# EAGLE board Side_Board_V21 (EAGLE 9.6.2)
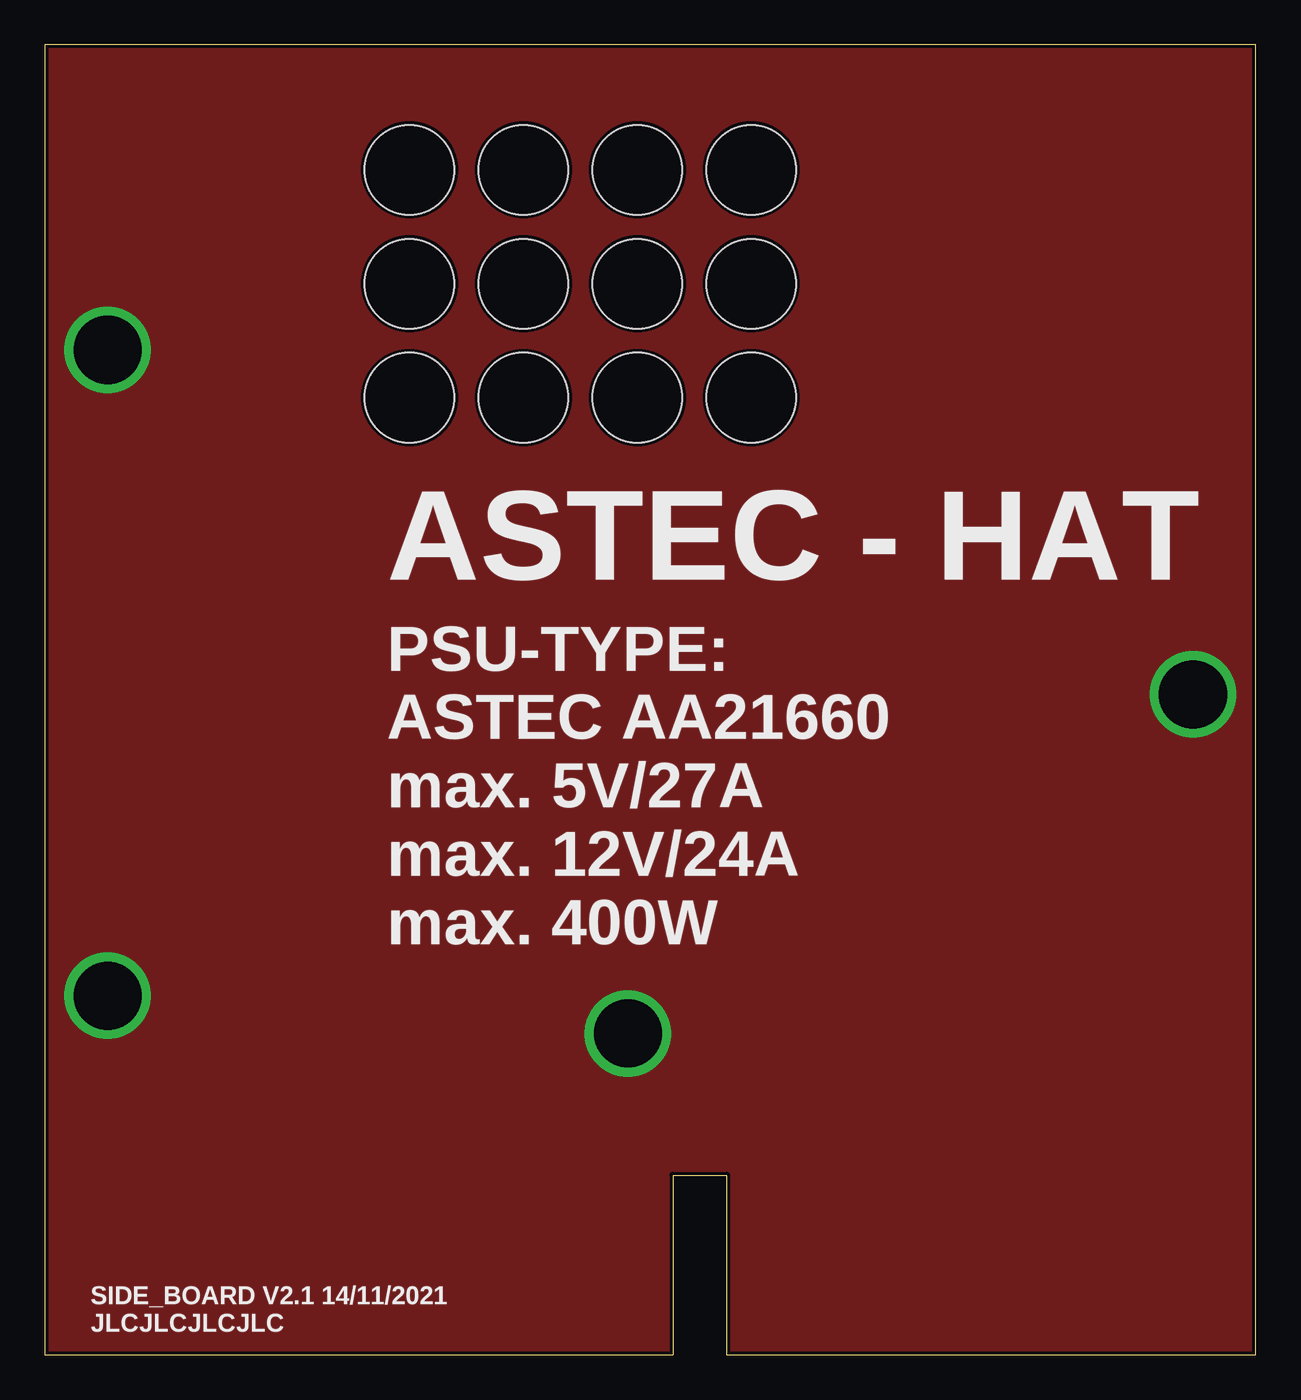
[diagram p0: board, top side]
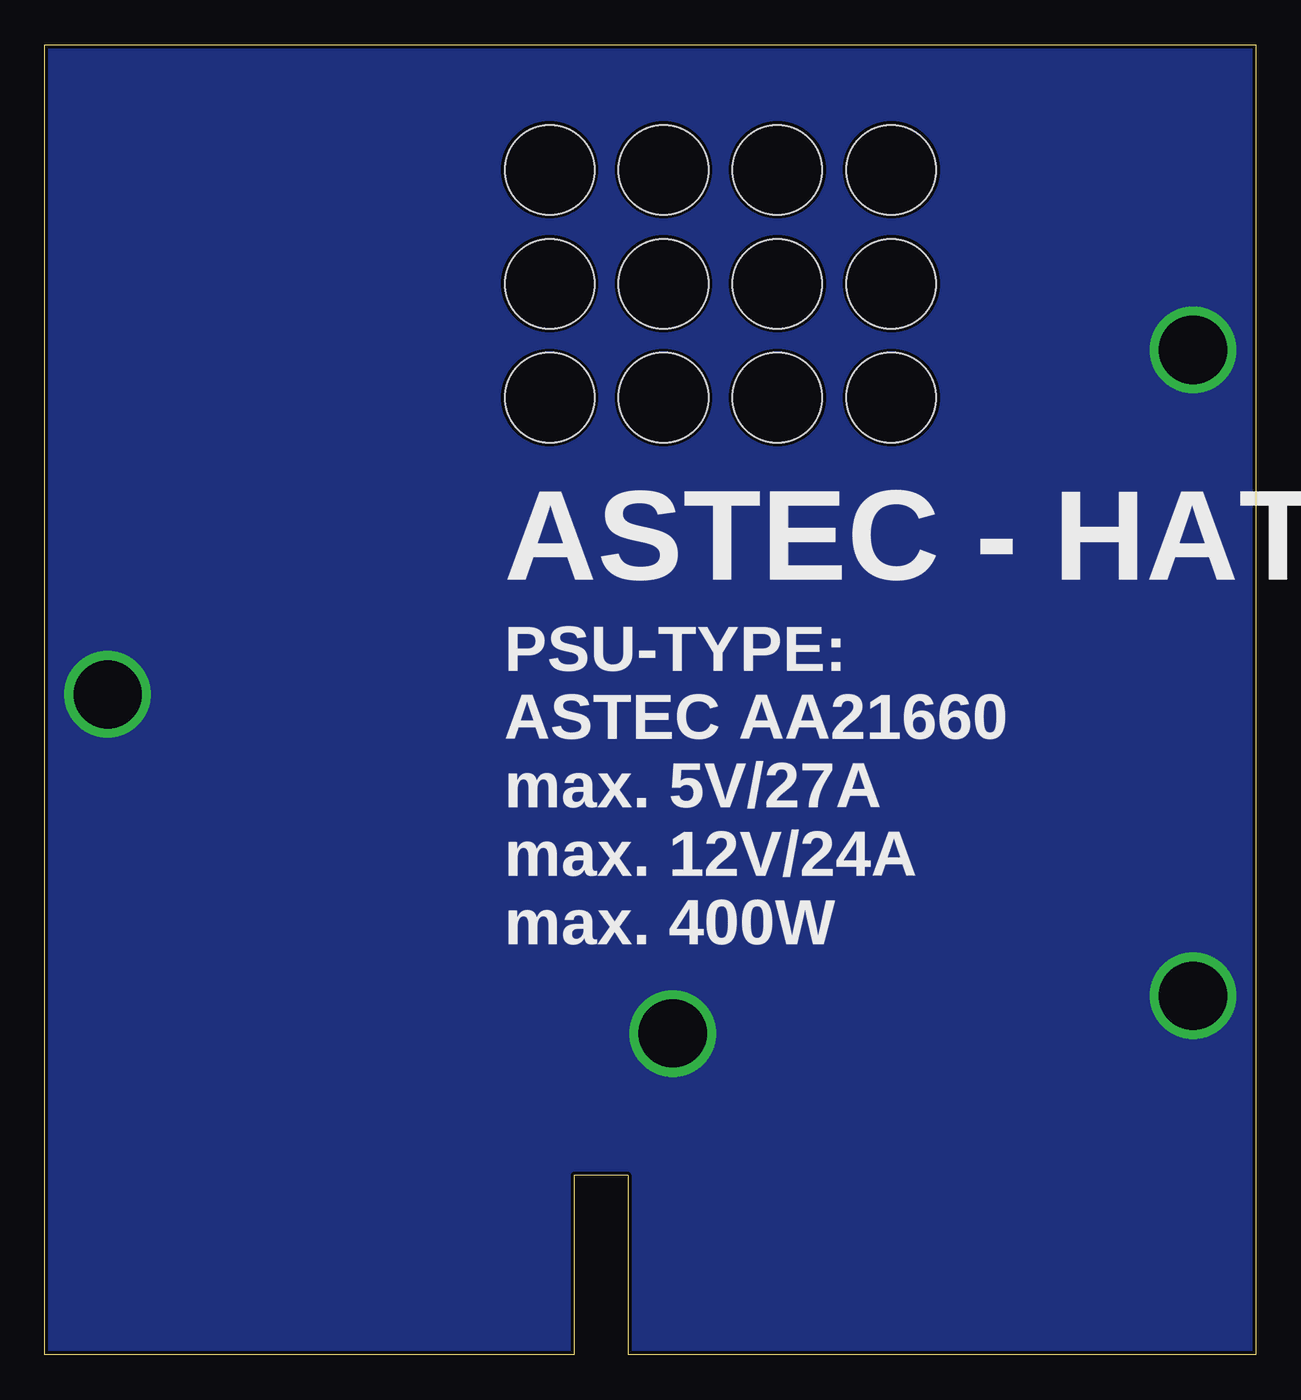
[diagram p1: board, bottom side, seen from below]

Size 67.5 x 73 mm. Coordinates in mm from the lower left corner, seen from the top.
Outline: 38,0 67.5,0 67.5,73 0,73 0,0 35,0 35,10 38,10 38,0
Copper layers (1*16): Top 0.035mm / dielectric 1.5mm / Bottom 0.035mm
Design rules "JLCPCB_2alyer": minimum track width 5mil, minimum drill 0.2mm, track to track 5mil, track to pad 0.2mm, pad to pad 0.2mm, via to via 0.2mm, smd to smd 5mil, copper to edge 0.2mm, drill to drill 0.5mm, minimum pad ring 0.13mm, minimum via ring 0.13mm, stop-mask expansion 0.05mm, vias tented up to drill 0mil, thermal gap 10mil
Holes 5 mm at 20.32,66.04 26.67,66.04 33.02,66.04 39.37,66.04 20.32,59.69 20.32,53.34 26.67,59.69 33.02,59.69 26.67,53.34 33.02,53.34 39.37,59.69 39.37,53.34

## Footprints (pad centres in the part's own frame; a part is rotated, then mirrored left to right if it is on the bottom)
M-PAD_3.8MM = drill 3.8 pad 4.4: P$1 0,0

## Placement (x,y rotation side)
P1  M-PAD_3.8MM  [M-PAD_3.8MM]  3.5,20 0 top
P2  M-PAD_3.8MM  [M-PAD_3.8MM]  3.5,56 0 top
P3  M-PAD_3.8MM  [M-PAD_3.8MM]  32.5,17.9 0 top
P4  M-PAD_3.8MM  [M-PAD_3.8MM]  64,36.8 0 top

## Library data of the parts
P1-P4 = Antec-Hood

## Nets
GND: P1.P$1 P2.P$1 P3.P$1 P4.P$1

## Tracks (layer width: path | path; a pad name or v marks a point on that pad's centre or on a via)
GND
  pour Top (no thermals): -2.54,74.93 -2.54,-5.08 71.12,-5.08 71.12,77.47 68.58,74.93 -1.27,74.93
  pour Bottom (no thermals): -3.81,77.47 -3.81,-7.62 -2.54,-8.89 72.39,-8.89 73.66,-7.62 73.66,77.47 72.39,78.74 -2.54,78.74

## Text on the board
tPlace: ASTEC - HAT | PSU-TYPE: / ASTEC AA21660 / max. 5V/27A / max. 12V/24A / max. 400W | SIDE_BOARD V2.1 14/11/2021 / JLCJLCJLCJLC
bPlace: ASTEC - HAT | PSU-TYPE: / ASTEC AA21660 / max. 5V/27A / max. 12V/24A / max. 400W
